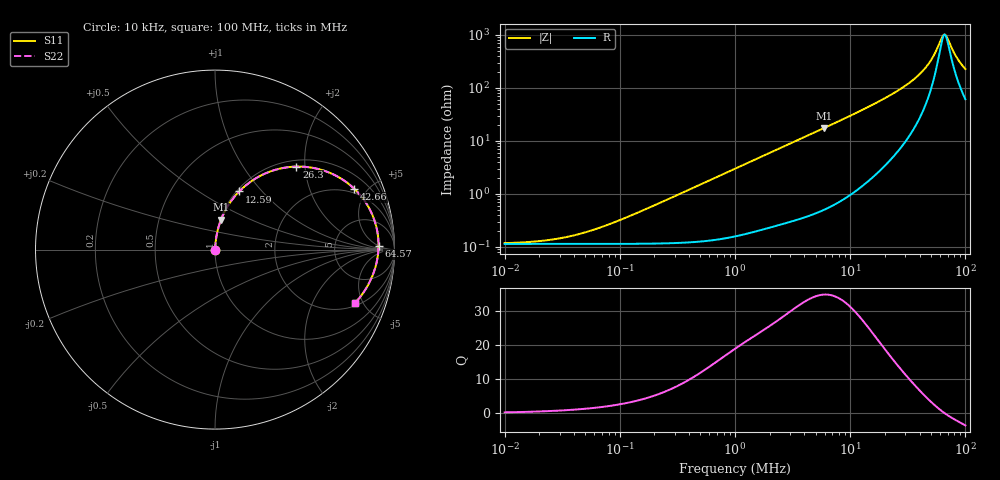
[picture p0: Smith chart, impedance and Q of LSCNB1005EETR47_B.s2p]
! LSCNB1005EETR47_B  S-PARAMETER MODEL  ( Standard Model )
! Model Generated by TAIYO YUDEN Corporation (http://www.ty-top.com)
! Version 1.0
! TAIYO YUDEN Control No. 190130
! Copyright(c) 2019 TAIYO YUDEN CO.,LTD. All Rights Reserved.
! Product Description (link to TY-COMPAS)
! https://ds.yuden.co.jp/TYCOMPAS/or/detail?pn=LSCNB1005EETR47MB&u=M
! Products Name : Inductors
! Characteristics :
!  Inductance : 0.47 [uH] , SRF(min) : - [Hz] , DC Resistance(max) : 140 [mOhm]
!  Rated Current : Saturation  1.2 [A] (dL = 30 [%]), Temp Rise  1.2 [A] (dT = 40 [degC])
!  Case Size : 1.0 x 0.5 / 0.039 x 0.02 [mm/inch] , Thickness : 0.55 / 0.022 [mm/inch]
!  (Conditions: Temperature = 25 [degC] , DC Bias Current = 0 [A])
! External Node Assignments :
!  1  o---GGG---o  2
! GND o---------o GND
! Frequency Range : 10kHz  -  100MHz  [ 402 STEP ]
# MHz S RI R 50
! Freq[MHz].  S11 Real  S11 Imag  S21 Real  S21 Imag  S12 Real  S12 Imag  S22 Real  S22 Imag
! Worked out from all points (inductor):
!   401 points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, 10 kHz to 100 MHz, reference 50 ohm
!   read as one part in series: L = 477 nH near 114.8 kHz
!   highest Q = 34.7 at 5.888 MHz (marker M1), where L = 467 nH
!   self-resonance near 66.2 MHz
!   S11 on the Smith chart (normalised r, x): 10 kHz: 1.00, +0.00; 12.59 MHz: 1.03, +0.76; 26.3 MHz: 1.13, +1.80; 42.66 MHz: 1.72, +4.12; 64.57 MHz: 20, +5; 100 MHz: 2.22, -4.36
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0.01  0.00114 0.000299  0.9989 -0.000299  0.9989 -0.000299  0.00114 0.000299
0.023442  0.00114 0.0007  0.9989 -0.0007  0.9989 -0.0007  0.00114 0.0007
0.046774  0.00114 0.0014  0.9989 -0.0014  0.9989 -0.0014  0.00114 0.0014
0.089125  0.00115 0.00266  0.9989 -0.00266  0.9989 -0.00266  0.00115 0.00266
0.218776  0.0012 0.00654  0.9988 -0.00654  0.9988 -0.00654  0.0012 0.00654
1  0.00246 0.0297  0.9975 -0.0297  0.9975 -0.0297  0.00246 0.0297
2.344229  0.00725 0.0684  0.9928 -0.0684  0.9928 -0.0684  0.00725 0.0684
4.677351  0.0223 0.1336  0.9777 -0.1336  0.9777 -0.1336  0.0223 0.1336
5.888437  0.0336 0.1663  0.9664 -0.1663  0.9664 -0.1663  0.0336 0.1663
12.58925  0.1348 0.3238  0.8652 -0.3238  0.8652 -0.3238  0.1348 0.3238
16.59587  0.2193 0.392  0.7807 -0.392  0.7807 -0.392  0.2193 0.392
21.87762  0.3451 0.447  0.6549 -0.447  0.6549 -0.447  0.3451 0.447
26.30268  0.4535 0.4626  0.5465 -0.4626  0.5465 -0.4626  0.4535 0.4626
33.88442  0.6248 0.4337  0.3752 -0.4337  0.3752 -0.4337  0.6248 0.4337
42.65795  0.7768 0.3381  0.2232 -0.3381  0.2232 -0.3381  0.7768 0.3381
51.28614  0.8679 0.2131  0.1321 -0.2131  0.1321 -0.2131  0.8679 0.2131
61.6595  0.9097 0.0605  0.0903 -0.0605  0.0903 -0.0605  0.9097 0.0605
64.56542  0.9111 0.0211  0.0889 -0.0211  0.0889 -0.0211  0.9111 0.0211
69.1831  0.9067 -0.0371  0.0933 0.0371  0.0933 0.0371  0.9067 -0.0371
83.17638  0.862 -0.1796  0.138 0.1796  0.138 0.1796  0.862 -0.1796
93.32543  0.8149 -0.2561  0.1851 0.2561  0.1851 0.2561  0.8149 -0.2561
100  0.7807 -0.2968  0.2193 0.2968  0.2193 0.2968  0.7807 -0.2968
